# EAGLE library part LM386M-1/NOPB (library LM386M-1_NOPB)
Audio Amplifiers LOW VLTG AUDIO PWR AMP
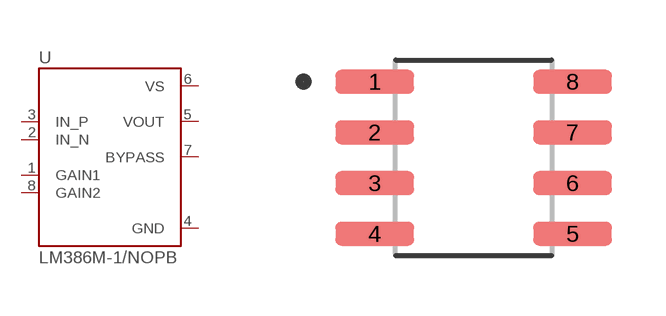
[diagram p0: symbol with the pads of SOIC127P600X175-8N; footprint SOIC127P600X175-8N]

Designator prefix U

## LM386M-1/NOPB (Availability: Unavailable; Description: Wide Input Voltage Low Power Audio Amplifier with Internal Gain 8-SOIC 0 to 70; MF: Texas Instruments; MP: LM386M-1; Package: SOIC-8 Texas Instruments; Price: None)  [SOIC127P600X175-8N]
1  GAIN1  pas
2  IN_N  in
3  IN_P  in
4  GND  pwr
5  VOUT  out
6  VS  pwr
7  BYPASS  out
8  GAIN2  pas

## Footprint SOIC127P600X175-8N (pad centres in mm)
smd 1.97 x 0.6: 1 -2.475,1.905; 2 -2.475,0.635; 3 -2.475,-0.635; 4 -2.475,-1.905; 5 2.475,-1.905; 6 2.475,-0.635; 7 2.475,0.635; 8 2.475,1.905

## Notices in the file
This work is licensed under a Creative Commons Attribution-ShareAlike 4.0 International License (CC BY-SA) with Design Exception 1.0
